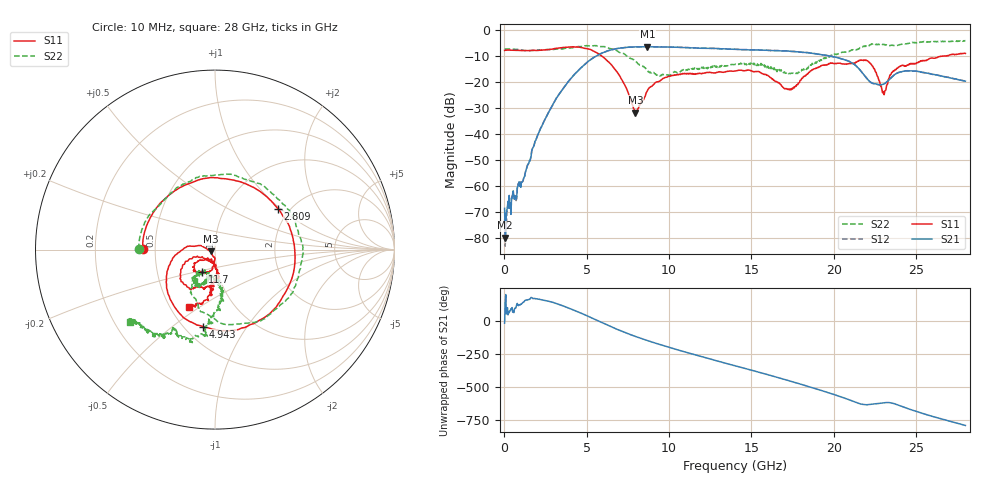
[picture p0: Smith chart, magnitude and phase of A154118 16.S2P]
!  2-Port S-parameters saved by WinCal
! VAR MeasName=S-Parameters (CALIBRATED_DATA) read from VNA (N5230A)
! VAR MeasDate=2015-9-10 14:35:31
! VAR NAME=A154118 16
! VAR FILENAME=A154118 16.S2P
! VAR DATE=2015-9-10 14:35:32
! VAR PHYS_PORTS=1,2
# Hz S DB R 50
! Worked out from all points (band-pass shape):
!   801 points, 10 MHz to 28 GHz, reference 50 ohm
!   highest |S21| = -6.55 dB at 8.687 GHz (marker M1); lowest = -80.0 dB at 44.99 MHz (marker M2)
!   |S21| within 3 dB of the highest: 5.755 GHz to 19.18 GHz (13.42 GHz wide, 108 % of centre)
!   lowest |S11| = -31.9 dB at 7.952 GHz (marker M3), VSWR 1.05, Z = 47.7 - j0.99 ohm
!   |S11| at or under -10 dB: 5.876 GHz to 26.9 GHz (21.02 GHz wide, 128 % of centre); 26.93273 GHz to 26.96041 GHz (27.68 MHz wide, 0.103 % of centre)
!   |S22| runs from -17.9 to -4.1 dB; largest |S21 - S12| = 0.007
!   S11 on the Smith chart (normalised r, x): 10 MHz: 0.43, +0.00; 2.809 GHz: 1.75, +0.96; 4.943 GHz: 0.61, -0.65; 11.7 GHz: 0.85, -0.21; 28 GHz: 0.62, -0.45
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1e7  -7.97 179.6  -68.73 -17.9  -73.07 -55.5  -7.48 179.7
4.49875e7  -7.93 178.1  -79.97 132.2  -83.25 78.4  -7.46 178.7
1.654412e9  -7.95 99.5  -46.83 175.0  -46.84 175.0  -8.05 133.4
2.809e9  -7.58 32.7  -30.32 143.7  -30.31 144.0  -7.67 95.4
3.6487e9  -6.79 -20.7  -21.91 108.5  -21.85 108.6  -7.25 60.5
4.698325e9  -6.87 -86.0  -14.43 55.2  -14.36 55.0  -6.46 12.4
4.943238e9  -7.25 -99.0  -13.01 42.5  -12.99 42.2  -6.21 -0.3
6.272762e9  -12.16 -166.3  -8.15 -34.0  -8.14 -34.2  -6.96 -65.8
7.952162e9  -31.87 -156.0  -6.62 -118.6  -6.62 -118.7  -11.95 -121.7
8.6869e9  -23.37 -94.1  -6.55 -150.3  -6.52 -150.5  -15.67 -124.3
9.351662e9  -19.95 -99.1  -6.66 -176.9  -6.63 -177.1  -17.85 -117.4
1.169582e10  -17.02 -119.7  -7.07 97.5  -7.02 97.0  -15.07 -102.8
1.4005e10  -15.94 -126.1  -7.57 18.6  -7.55 18.1  -13.41 -112.6
1.54045e10  -16.05 -142.2  -7.81 -28.8  -7.77 -29.4  -13.63 -117.8
1.729382e10  -23.17 -114.4  -8.30 -95.3  -8.26 -96.1  -16.86 -112.7
1.869332e10  -15.36 -87.9  -9.09 -147.6  -9.10 -148.1  -12.95 -80.9
2.065262e10  -13.26 -115.2  -11.55 133.7  -11.57 132.9  -8.64 -90.7
2.191218e10  -11.84 -134.5  -18.00 83.6  -18.02 82.8  -6.28 -94.9
2.299679e10  -23.77 -123.1  -21.03 96.8  -21.10 96.5  -5.61 -114.6
2.334666e10  -18.83 -82.8  -19.35 99.3  -19.35 99.2  -6.17 -116.8
2.450125e10  -13.70 -96.3  -15.82 53.7  -15.78 53.0  -5.34 -119.8
2.8e10  -9.15 -114.3  -19.79 -74.1  -19.86 -74.8  -4.15 -139.6
